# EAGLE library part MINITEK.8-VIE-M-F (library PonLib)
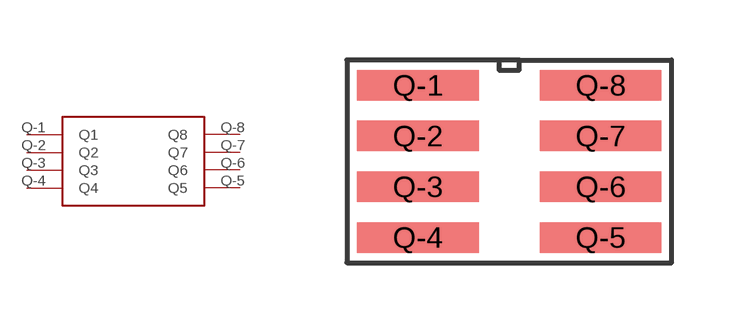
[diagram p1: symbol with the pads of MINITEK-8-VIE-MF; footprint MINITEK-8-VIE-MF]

Designator prefix -

## MINITEK.8-VIE-M-F  [MINITEK-8-VIE-MF]
Q-1  Q1
Q-2  Q2
Q-3  Q3
Q-4  Q4
Q-5  Q5
Q-6  Q6
Q-7  Q7
Q-8  Q8

## Footprint MINITEK-8-VIE-MF (pad centres in mm)
smd 3.048 x 0.762: Q-1 -2.286,1.905; Q-2 -2.286,0.635; Q-3 -2.286,-0.635; Q-4 -2.286,-1.905; Q-5 2.286,-1.905; Q-6 2.286,-0.635; Q-7 2.286,0.635; Q-8 2.286,1.905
